TYPE IGS_IN :
STRUCT
	//C32	EL3164	4AI	0-10V
	C32		:ARRAY [1..4] OF INT;
	
	
	//C33	EL3164	4AI	0-10V
	C33		:ARRAY [1..4] OF INT;
	
	
	//C34	EL3164	4AI	0-10V
	C34		:ARRAY [1..4] OF INT;
	
	
	//C35	EL3154	4AI	4-20mA
	C35		:ARRAY [1..4] OF INT;
	
	
	//C36	EL1889 16DI
	C36		:ARRAY [1..16] OF BOOL;
	
	
	
	//C37	EL1889 16DI
	C37		:ARRAY [1..16] OF BOOL;
	
	
	//C38	EL1904	4SDI
	C38		:ARRAY [1..4] OF BOOL;
	
	//C39	EL1904	4SDI
	C39		:ARRAY [1..4] OF BOOL;
	
	//C40	EL3318	8TC
	C40		:ARRAY [1..8] OF INT;
	
	//C41	EL9410	POWER MODULE
		
	
END_STRUCT
END_TYPE
